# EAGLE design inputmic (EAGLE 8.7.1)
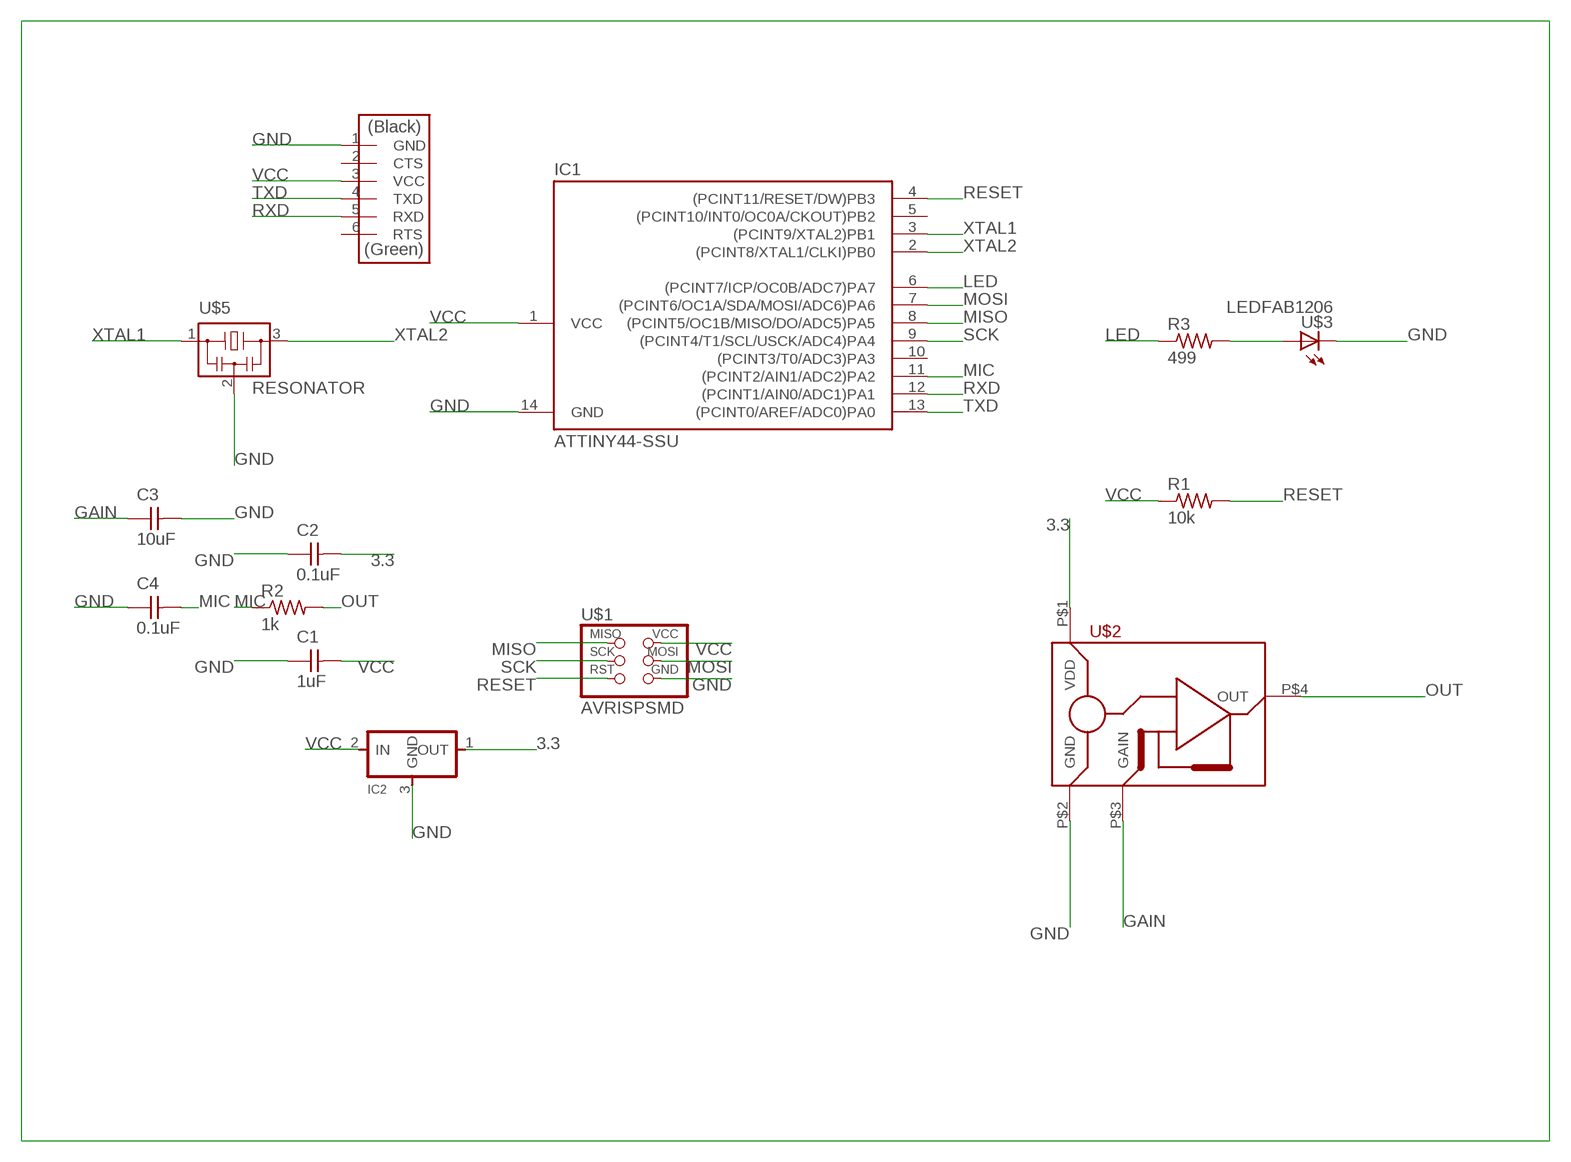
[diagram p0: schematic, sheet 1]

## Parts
C1  1uF  CAP-UNPOLARIZEDFAB  [C1206FAB]
C2  0.1uF  CAP-UNPOLARIZEDFAB  [C1206FAB]
C3  10uF  CAP-UNPOLARIZEDFAB  [C1206FAB]
C4  0.1uF  CAP-UNPOLARIZEDFAB  [C1206FAB]
IC1  ATTINY44-SSU  [SOIC14]
IC2  REGULATORSOT23  [SOT23]
R1  10k  RES-US1206FAB  [R1206FAB]
R2  1k  RES-US1206FAB  [R1206FAB]
R3  499  RES-US1206FAB  [R1206FAB]
U$1  AVRISPSMD  [2X03SMD]
U$2  MEMS_MIC_SPU0414HR5H-SB  [CSP-4PIN]
U$3  LEDFAB1206  [LED1206FAB]
U$4  FTDI-SMD-HEADER  [1X06SMD]
U$5  RESONATOR  [EFOBM]

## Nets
3.3: C2.2 IC2.1(OUT) U$2.P$1(VDD)
GAIN: C3.1 U$2.P$3(GAIN)
GND: C1.1 C2.1 C3.2 C4.1 IC1.14(GND) IC2.3(GND) U$1.6(GND) U$2.P$2(GND) U$3.2(C) U$4.1(GND) U$5.2
LED: IC1.6((PCINT7/ICP/OC0B/ADC7)PA7) R3.1
MIC: C4.2 IC1.11((PCINT2/AIN1/ADC2)PA2) R2.1
MISO: IC1.8((PCINT5/OC1B/MISO/DO/ADC5)PA5) U$1.1(MISO)
MOSI: IC1.7((PCINT6/OC1A/SDA/MOSI/ADC6)PA6) U$1.4(MOSI)
N$6: R3.2 U$3.1(A)
OUT: R2.2 U$2.P$4(OUT)
RESET: IC1.4((PCINT11/RESET/DW)PB3) R1.2 U$1.5(RST)
RXD: IC1.12((PCINT1/AIN0/ADC1)PA1) U$4.5(RXD)
SCK: IC1.9((PCINT4/T1/SCL/USCK/ADC4)PA4) U$1.3(SCK)
TXD: IC1.13((PCINT0/AREF/ADC0)PA0) U$4.4(TXD)
VCC: C1.2 IC1.1(VCC) IC2.2(IN) R1.1 U$1.2(VCC) U$4.3(VCC)
XTAL1: IC1.3((PCINT9/XTAL2)PB1) U$5.1
XTAL2: IC1.2((PCINT8/XTAL1/CLKI)PB0) U$5.3
Unconnected: IC1.5((PCINT10/INT0/OC0A/CKOUT)PB2) IC1.10((PCINT3/T0/ADC3)PA3) U$4.2(CTS) U$4.6(RTS)

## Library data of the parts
C1-C4 = fab:CAP-UNPOLARIZED
IC1 = fab:ATTINY44
IC2 = fab:REGULATOR
R1-R3 = fab:RES-US: Resistor (US Symbol)
U$1 = fab:AVRISP
U$2 = fab:MEMS_MIC_SPU0414HR5H-SB
U$3 = fab:LED: LED
U$4 = fab:FTDI-SMD-HEADER
U$5 = fab:RESONATOR

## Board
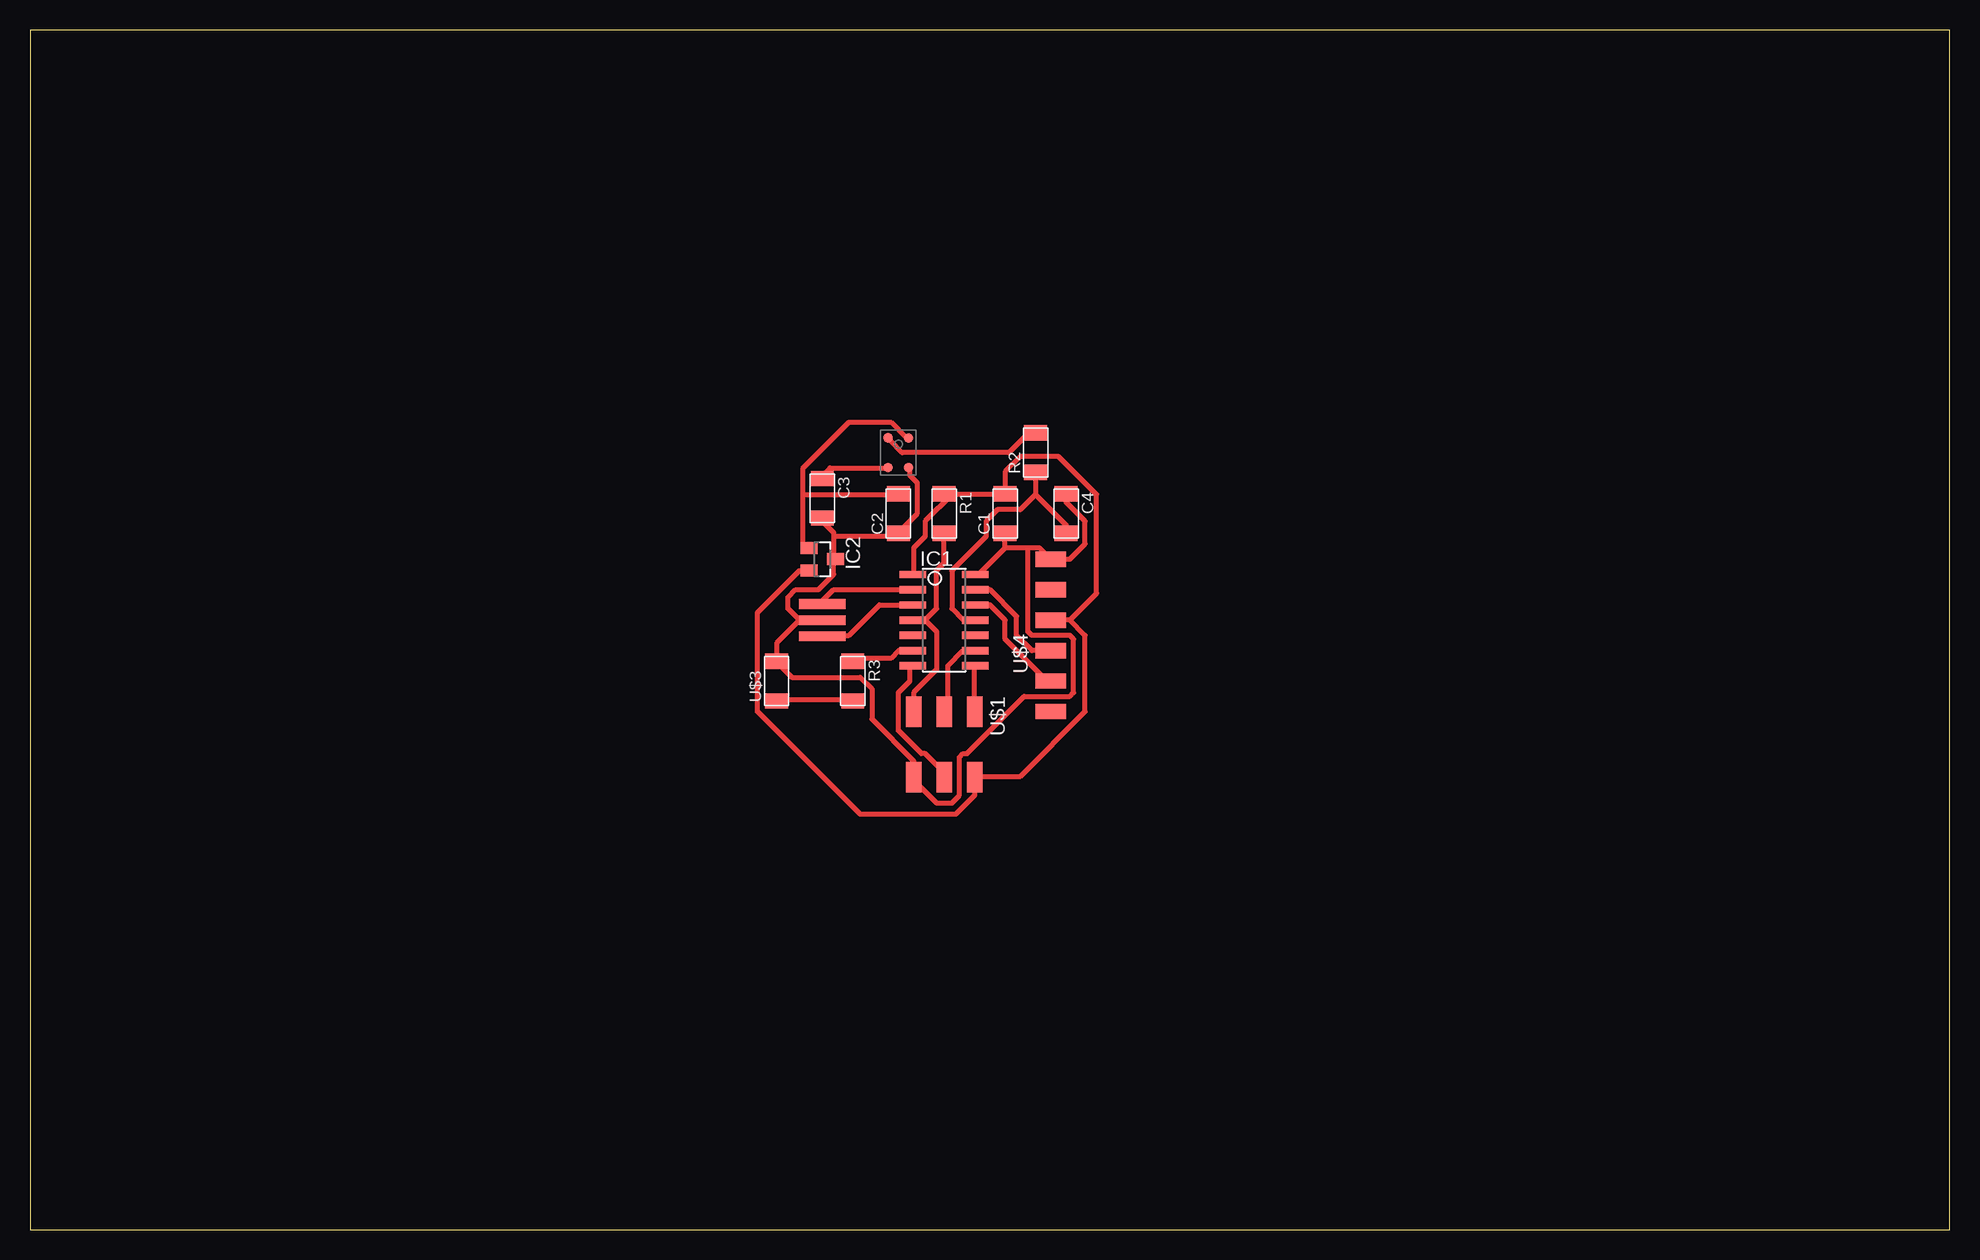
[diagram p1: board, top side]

Size 160 x 100 mm. Coordinates in mm from the lower left corner, seen from the top.
Outline: 0,0 160,0 160,100 0,100 0,0
Copper layers (1*16): Top 0.035mm / dielectric 1.5mm / Bottom 0.035mm
Design rules "default *": minimum track width 16mil, minimum drill 0.35mm, track to track 16mil, track to pad 16mil, pad to pad 16mil, via to via 16mil, smd to smd 16mil, copper to edge 40mil, drill to drill 6mil, minimum pad ring 10mil, minimum via ring 8mil, stop-mask expansion 4mil, vias tented up to drill 0mil, thermal gap 10mil

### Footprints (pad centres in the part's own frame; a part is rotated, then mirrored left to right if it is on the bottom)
C1206FAB = smd 1.27 x 1.905: 1 -1.651,0; 2 1.651,0
SOIC14 = smd 0.61 x 2.21: 1 -3.81,-2.603; 2 -2.54,-2.603; 3 -1.27,-2.603; 4 0,-2.603; 5 1.27,-2.603; 6 2.54,-2.603; 7 3.81,-2.603; 8 3.81,2.603; 9 2.54,2.603; 10 1.27,2.603; 11 0,2.603; 12 -1.27,2.603; 13 -2.54,2.603; 14 -3.81,2.603
SOT23 = smd 1 x 1.4: 1 -0.95,-1.1; 2 0.95,-1.1; 3 0,1.1
R1206FAB = smd 1.27 x 1.905: 1 -1.651,0; 2 1.651,0
2X03SMD = smd 2.54 x 1.27: 1 -2.54,2.54; 2 2.92,2.54; 3 -2.54,0; 4 2.92,0; 5 -2.54,-2.54; 6 2.92,-2.54
CSP-4PIN = smd 0.8 x 0.8: P$1 0.855,1.215; P$2 0.85,-1.23; P$3 -0.85,-1.23; P$4 -0.85,1.23
LED1206FAB = smd 1.27 x 1.905: 1 -1.651,0; 2 1.651,0
1X06SMD = smd 2.54 x 1.27: 1 0,6.35; 2 0,3.81; 3 0,1.27; 4 0,-1.27; 5 0,-3.81; 6 0,-6.35
EFOBM = smd 0.8 x 3.9: 1 -1.35,0; 2 0,0; 3 1.35,0

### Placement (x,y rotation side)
C1  81.28,59.69 90 top
C2  72.39,59.69 90 top
C3  66.04,60.96 270 top
C4  86.36,59.69 270 top
IC1  76.2,50.8 270 top
IC2  66.04,55.88 270 top
R1  76.2,59.69 270 top
R2  83.82,64.77 90 top
R3  68.58,45.72 270 top
U$1  76.2,40.64 270 top
U$2  72.39,64.77 0 top
U$3  62.23,45.72 90 top
U$4  85.09,49.53 0 top
U$5  66.04,50.8 90 top

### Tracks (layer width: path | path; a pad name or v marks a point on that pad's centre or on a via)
3.3
  Top 0.406: 64.45,61.28 64.45,57.15 64.77,56.83 IC2.1 | 64.45,61.28 64.45,63.5 68.26,67.31 71.75,67.31 73.03,66.04 U$2.P$1 | 64.45,61.28 72.39,61.28 C2.2
GAIN
  Top 0.406: U$2.P$3 71.44,63.5 66.67,63.5 66.04,62.87 C3.1
GND
  Top 0.406: 81.28,56.83 C1.1 | 81.28,56.83 79.06,54.61 IC1.14 | C4.1 86.36,60.64 87.95,59.05 87.95,57.15 86.68,55.88 U$4.1 84.14,56.83 83.19,56.83 | 83.19,56.83 81.28,56.83 | 66.99,57.78 66.99,58.1 66.04,59.05 C3.2 | 66.99,57.78 66.99,55.88 | U$2.P$2 73.34,63.5 73.34,62.87 73.98,62.23 73.98,59.69 72.39,58.1 C2.1 72.39,57.78 66.99,57.78 | 64.14,50.8 62.23,48.9 U$3.2 62.23,47.31 63.5,46.04 69.22,46.04 70.17,45.09 70.17,42.55 73.66,39.05 U$1.6 73.66,37.47 75.56,35.56 76.83,35.56 77.47,36.2 77.47,39.37 77.79,39.69 78.11,39.69 82.87,44.45 86.68,44.45 87,44.77 87,49.21 86.68,49.53 83.5,49.53 83.19,49.85 83.19,56.83 | 66.99,55.88 66.99,54.61 65.72,53.34 63.82,53.34 63.18,52.7 63.18,51.75 64.14,50.8 | 66.99,55.88 IC2.3 | 64.14,50.8 U$5.2
LED
  Top 0.406: IC1.6 72.39,48.26 71.75,47.62 68.58,47.62 R3.1
MIC
  Top 0.406: C4.2 86.36,58.74 83.82,61.28 | R2.1 83.82,61.28 | IC1.11 77.79,50.8 76.83,51.75 76.83,54.93 79.69,57.78 79.69,59.05 80.64,60.01 82.55,60.01 83.82,61.28
MISO
  Top 0.406: U$1.1 78.74,46.99 IC1.8
MOSI
  Top 0.406: U$1.4 76.2,38.1 74.61,39.69 74.3,39.69 72.39,41.59 72.39,44.77 73.34,45.72 73.34,46.99 IC1.7
N$6
  Top 0.406: U$3.1 62.23,44.13 68.58,44.13 R3.2
OUT
  Top 0.406: U$2.P$4 71.75,65.72 72.71,64.77 81.6,64.77 83.19,66.36 83.82,66.36 R2.2
RESET
  Top 0.406: R1.2 76.2,55.56 75.56,54.93 75.56,51.75 74.61,50.8 | 74.61,50.8 IC1.4 73.66,50.8 | U$1.5 73.66,44.77 75.56,46.67 75.56,49.85 74.61,50.8
RXD
  Top 0.406: IC1.12 80.01,52.07 81.28,50.8 81.28,49.21 84.77,45.72 U$4.5
SCK
  Top 0.406: IC1.9 77.79,48.26 76.52,46.99 76.52,43.5 U$1.3
TXD
  Top 0.406: IC1.13 80.01,53.34 82.23,51.12 82.23,49.53 83.5,48.26 U$4.4
VCC
  Top 0.406: 76.83,61.28 81.28,61.28 C1.2 81.28,63.18 82.55,64.45 85.72,64.45 88.9,61.28 88.9,53.02 86.68,50.8 | 76.83,61.28 76.2,61.28 R1.1 76.83,61.28 | 76.83,61.28 74.61,59.05 74.61,57.78 73.66,56.83 73.66,54.61 IC1.1 | IC2.2 64.77,54.93 64.14,54.93 60.64,51.44 60.64,43.18 69.22,34.61 77.15,34.61 78.74,36.2 U$1.2 78.74,37.78 82.55,37.78 87.95,43.18 87.95,49.53 86.68,50.8 | 86.68,50.8 U$4.3
XTAL1
  Top 0.406: IC1.3 70.8,52.07 68.26,49.53 66.04,49.53 U$5.1
XTAL2
  Top 0.406: IC1.2 66.99,53.34 66.04,52.39 U$5.3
